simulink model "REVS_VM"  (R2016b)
settings: Solver=ode3  StartTime=REVS.sim_start_time_secs  StopTime=Inf  FixedStep=REVS.sim_step_time_secs  MaxStep=REVS.sim_step_time_secs  EnableMultiTasking=on
StopFcn:
  | postproc_datalog;
  | postproc_audit;
  | postproc_result;
model workspace (MATLAB code in the model file):
  other statements: REVS_setup_variants
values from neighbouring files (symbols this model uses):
  accessory = class_accessory_data    [class_test_data.m]
  battery = class_battery_data    [class_accessory_data.m]    (also in class_REVS_electric.m = class_REVS_battery)
  brake = struct(	'max_torque_Nm',[], 						'proportion_norm',1.0, 						'inertia_kgm2',0.0)    [class_REVS_drive_axle.m]
  engine = class_engine_data    [class_test_data.m]
  final_drive = struct(	'gear_ratio',[], 								'efficiency_norm',[], 								'inertia_kgm2',[] )    [class_REVS_drive_axle.m]
  gear = class_REVS_gearbox    [class_REVS_AT_transmission.m]
  tire = struct(	'radius_m',[], 						'rolling_resistance_coefficient',0, 						'vehicle_weight_norm',1.0,  						'wheel_slip_torque_Nm',[],  						'inertia_kgm2',0.0)    [class_REVS_drive_axle.m]
  torque_converter = class_REVS_torque_converter    [class_REVS_AT_transmission.m]
  transmission = class_transmission_data    [class_test_data.m]
  vehicle = class_vehicle_data    [class_test_data.m]
undefined symbols (not defined in the file or in its folder): alternator, ambient, controls, convert, DelayTimeSecs, drive_cycle, driver, electric, gear_strategy, InitialCondition, InitialValue, LoadSource, LookupStructure, MultiplyPosInputs, Normalize, NumPhases, REVS, SpeedSource, starter, tableshift, UpperSaturationLimit, Value, VerboseLevel, VerboseSignal
libraries: simulink x153
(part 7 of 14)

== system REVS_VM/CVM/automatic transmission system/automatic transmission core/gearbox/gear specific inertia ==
  engage : Inport
  cmd_gear_num : Inport  Port=2
  iner_spd_out_radps : Inport  Port=3
  1-D Lookup Table : Lookup_n-D  NumberOfTableDimensions=1  BreakpointsForDimension1=gear.number  Table=gear.inertia_kgm2  InternalRulePriority=Speed  RndMeth=Simplest
  Derivative : Derivative
  Detect Decrease : simulink/Logic and Bit Operations/Detect Decrease  vinit=0.0  InputProcessing=Inherited  OutDataTypeStr=boolean
  Gain : Gain  Gain=.5/1000
  Gain1 : Gain  Gain=0.5
  Inertia Mech E&P Nm radps : Subsystem
  Memory : Memory
  Memory1 : Memory
  Product : Product  Inputs=3
  Product1 : Product
  Product4 : Product
  Product5 : Product
  Saturation : Saturate  UpperLimit=inf  LowerLimit=0
  Sum : Sum  Inputs=|++
  inertia KE loss : Subsystem
  iner_trq_out_Nm : Outport
  iner_out_kgm2 : Outport  Port=2
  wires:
  cmd_gear_num/1 -> 1-D Lookup Table/1
  Memory1/1 -> Sum/2
  Sum/1 -> inertia KE loss/1(Var), Memory1/1
  Gain1/1 -> Inertia Mech E&P Nm radps/1(trq_Nm)
  Product5/1 -> Gain1/1, iner_trq_out_Nm/1
  Product4/1 -> iner_out_kgm2/1, Product/1, Derivative/1
  iner_spd_out_radps/1 -> Product5/2, Inertia Mech E&P Nm radps/2(spd_radps), Product/2, Product/3
  Memory/1 -> Product1/1
  Detect Decrease/1 -> Product1/2
  Product/1 -> Gain/1
  Gain/1 -> Memory/1
  engage/1 -> Product4/1, Detect Decrease/1
  Derivative/1 -> Saturation/1
  Saturation/1 -> Product5/1
  1-D Lookup Table/1 -> Product4/2
  Product1/1 -> Sum/1

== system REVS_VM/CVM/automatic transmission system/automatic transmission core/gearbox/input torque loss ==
  bus : Inport
  Bus Selector : BusSelector  OutputSignals=gb.gb_cmd_gear,gb_spd_in_radps,ctrl.gb_line_press_bar
  Lookup : Lookup_n-D  NumberOfTableDimensions=10  BreakpointsForDimension1=LookupStructure.axis_1.breakpoints  BreakpointsForDimension2=LookupStructure.axis_2.breakpoints  BreakpointsForDimension3=LookupStructure.axis_3.breakpoints  BreakpointsForDimension4=LookupStructure.axis_4.breakpoints  BreakpointsForDimension5=LookupStructure.axis_5.breakpoints  BreakpointsForDimension6=LookupStructure.axis_6.breakpoints  BreakpointsForDimension7=LookupStructure.axis_7.breakpoints  BreakpointsForDimension8=LookupStructure.axis_8.breakpoints  BreakpointsForDimension9=LookupStructure.axis_9.breakpoints  BreakpointsForDimension10=LookupStructure.axis_10.breakpoints  IndexSearchMethod=Linear search  BeginIndexSearchUsingPreviousIndexResult=on  Table=LookupStructure.table  InternalRulePriority=Speed  RndMeth=Simplest  SupportTunableTableSize=on  MaximumIndicesForEachDimension=LookupStructure.table_size
  out : Outport
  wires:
  bus/1 -> Bus Selector/1
  Lookup/1 -> out/1

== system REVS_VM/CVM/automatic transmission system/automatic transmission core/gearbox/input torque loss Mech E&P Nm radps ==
  trq_Nm : Inport
  spd_radps : Inport  Port=2
  Compare To Constant : simulink/Logic and Bit Operations/Compare To Constant  relop=>=  const=1  OutDataTypeStr=boolean
  Constant : Constant  Value=VerboseSignal
  Subsystem : Subsystem
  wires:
  trq_Nm/1 -> Subsystem/1(trq_Nm)
  spd_radps/1 -> Subsystem/2(spd_radps)
  Compare To Constant/1 -> Subsystem/Enable
  Constant/1 -> Compare To Constant/1

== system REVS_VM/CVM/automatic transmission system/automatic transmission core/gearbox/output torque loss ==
  bus : Inport
  Bus Selector : BusSelector  OutputSignals=gb.gb_cmd_gear,gb_spd_in_radps,ctrl.gb_line_press_bar
  Lookup : Lookup_n-D  NumberOfTableDimensions=10  BreakpointsForDimension1=LookupStructure.axis_1.breakpoints  BreakpointsForDimension2=LookupStructure.axis_2.breakpoints  BreakpointsForDimension3=LookupStructure.axis_3.breakpoints  BreakpointsForDimension4=LookupStructure.axis_4.breakpoints  BreakpointsForDimension5=LookupStructure.axis_5.breakpoints  BreakpointsForDimension6=LookupStructure.axis_6.breakpoints  BreakpointsForDimension7=LookupStructure.axis_7.breakpoints  BreakpointsForDimension8=LookupStructure.axis_8.breakpoints  BreakpointsForDimension9=LookupStructure.axis_9.breakpoints  BreakpointsForDimension10=LookupStructure.axis_10.breakpoints  IndexSearchMethod=Linear search  BeginIndexSearchUsingPreviousIndexResult=on  Table=LookupStructure.table  DiagnosticForOutOfRangeInput=Warning  InternalRulePriority=Speed  RndMeth=Simplest  SupportTunableTableSize=on  MaximumIndicesForEachDimension=LookupStructure.table_size
  out : Outport
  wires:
  bus/1 -> Bus Selector/1
  Lookup/1 -> out/1

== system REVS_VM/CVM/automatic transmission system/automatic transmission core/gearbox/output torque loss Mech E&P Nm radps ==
  trq_Nm : Inport
  spd_radps : Inport  Port=2
  Compare To Constant : simulink/Logic and Bit Operations/Compare To Constant  relop=>=  const=1  OutDataTypeStr=boolean
  Constant : Constant  Value=VerboseSignal
  Subsystem : Subsystem
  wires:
  trq_Nm/1 -> Subsystem/1(trq_Nm)
  spd_radps/1 -> Subsystem/2(spd_radps)
  Compare To Constant/1 -> Subsystem/Enable
  Constant/1 -> Compare To Constant/1

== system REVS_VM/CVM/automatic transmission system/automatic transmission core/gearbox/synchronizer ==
  engage : Inport
  sync_trq_in_Nm : Inport  Port=2
  sync_iner_in_kgm2 : Inport  Port=3
  sync_spd_out_radps : Inport  Port=4
  " clutch input speed integrator (integrate when slipping)" : Integrator  ExternalReset=falling  InitialConditionSource=external  LimitOutput=on  UpperSaturationLimit=Inf  LowerSaturationLimit=0
  Clutch Speed Disengaged : Switch  Threshold=1
  IC1 : InitialCondition  Value=0
  Product : Product
  Product2 : Product  Inputs=*/
  Product3 : Product
  Subsystem : Subsystem
  Sum1 : Sum  Inputs=+-|
  Sum2 : Sum  Inputs=+-|
  Torque SW : Switch  Threshold=1
  engage target speed calc : Subsystem
  synchro limit torque : Subsystem
  to datalog with base name : Subsystem
  to datalog with base name1 : Subsystem
  to datalog with base name2 : Subsystem
  sync_trq_out_Nm : Outport
  sync_iner_out_kgm2 : Outport  Port=2
  sync_spd_in_radps : Outport  Port=3
  sync_lockup : Outport  Port=4
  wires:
  Product2/1 -> " clutch input speed integrator (integrate when slipping)"/1
  synchro limit torque/1(lim_transmit_torque_Nm) -> Sum1/2, to datalog with base name1/1(Var), Torque SW/3
  Product3/1 -> sync_iner_out_kgm2/1
  Torque SW/1 -> sync_trq_out_Nm/1
  Product/1 -> Sum2/2, to datalog with base name2/1(Var)
  " clutch input speed integrator (integrate when slipping)"/1 -> Clutch Speed Disengaged/3
  sync_trq_in_Nm/1 -> Sum2/1, Sum1/1, Torque SW/1
  IC1/1 -> " clutch input speed integrator (integrate when slipping)"/3
  sync_iner_in_kgm2/1 -> Product3/1, Product/2, Product2/2
  engage target speed calc/1(engage_accel_radps2) -> Product/1
  Sum2/1 -> synchro limit torque/2("req_transmit_torque_Nm ")
  Sum1/1 -> Product2/1
  engage/1 -> engage target speed calc/1(engage), Subsystem/1(engage), synchro limit torque/1(engage)
  sync_spd_out_radps/1 -> Subsystem/2(spd_out), synchro limit torque/4(output_speed_radps), IC1/1, engage target speed calc/2(final_spd_radps), Clutch Speed Disengaged/1
  Clutch Speed Disengaged/1 -> sync_spd_in_radps/1, synchro limit torque/3(input_speed_radps), Subsystem/3(spd_in), engage target speed calc/3(current_spd_radps)
  Subsystem/1(lockup) -> to datalog with base name/1(Var), " clutch input speed integrator (integrate when slipping)"/2, sync_lockup/1, Clutch Speed Disengaged/2, Product3/2, Torque SW/2

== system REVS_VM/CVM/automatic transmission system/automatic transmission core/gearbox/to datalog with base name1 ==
  Var : Inport
  Constant : Constant  Value=VerboseSignal
  Constant1 : Constant  Value=VerboseLevel
  Relational Operator : RelationalOperator  OutDataTypeStr=boolean  ZeroCross=off
  Subsystem : Subsystem
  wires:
  Constant1/1 -> Relational Operator/2
  Relational Operator/1 -> Subsystem/Enable
  Constant/1 -> Relational Operator/1
  Var/1 -> Subsystem/1(Var)

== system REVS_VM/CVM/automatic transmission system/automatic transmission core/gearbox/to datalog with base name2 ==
  Var : Inport
  Constant : Constant  Value=VerboseSignal
  Constant1 : Constant  Value=VerboseLevel
  Relational Operator : RelationalOperator  OutDataTypeStr=boolean  ZeroCross=off
  Subsystem : Subsystem
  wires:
  Constant1/1 -> Relational Operator/2
  Relational Operator/1 -> Subsystem/Enable
  Constant/1 -> Relational Operator/1
  Var/1 -> Subsystem/1(Var)

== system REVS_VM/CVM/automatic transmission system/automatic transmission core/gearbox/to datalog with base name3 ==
  Var : Inport
  Constant : Constant  Value=VerboseSignal
  Constant1 : Constant  Value=VerboseLevel
  Relational Operator : RelationalOperator  OutDataTypeStr=boolean  ZeroCross=off
  Subsystem : Subsystem
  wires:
  Constant1/1 -> Relational Operator/2
  Relational Operator/1 -> Subsystem/Enable
  Constant/1 -> Relational Operator/1
  Var/1 -> Subsystem/1(Var)

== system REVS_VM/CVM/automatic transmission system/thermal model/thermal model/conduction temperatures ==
  bus : Inport
  Bus Selector : BusSelector  OutputSignals=signal1,bus.signal2  OutputAsBus=on
  Reshape : Reshape
  out : Outport
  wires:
  Bus Selector/1 -> Reshape/1
  bus/1 -> Bus Selector/1
  Reshape/1 -> out/1

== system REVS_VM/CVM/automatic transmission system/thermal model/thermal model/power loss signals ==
  bus : Inport
  Bus Creator : BusCreator  Inputs=10
  Bus Creator1 : BusCreator  Inputs=2
  Bus Selector : BusSelector  OutputSignals=var_sigs.var_sig1  OutputAsBus=on
  Data Type Conversion : DataTypeConversion  OutDataTypeStr=double
  Display : Display
  Fcn : Fcn
  Variable {1..10} (10 alike) : Constant  Value=nan
  out : Outport
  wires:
  Data Type Conversion/1 -> Fcn/1
  Bus Selector/1 -> Data Type Conversion/1, Display/1
  Bus Creator1/1 -> Bus Selector/1
  Fcn/1 -> out/1
  bus/1 -> Bus Creator1/1  "system_bus"
  Bus Creator/1 -> Bus Creator1/2  "var_sigs"
  Variable 1/1 -> Bus Creator/1  "var_sig1"
  Variable 2/1 -> Bus Creator/2  "var_sig2"
  Variable 3/1 -> Bus Creator/3  "var_sig3"
  Variable 4/1 -> Bus Creator/4  "var_sig4"
  Variable 5/1 -> Bus Creator/5  "var_sig5"
  Variable 6/1 -> Bus Creator/6  "var_sig6"
  Variable 7/1 -> Bus Creator/7  "var_sig7"
  Variable 8/1 -> Bus Creator/8  "var_sig8"
  Variable 9/1 -> Bus Creator/9  "var_sig9"
  Variable 10/1 -> Bus Creator/10  "var_sig10"

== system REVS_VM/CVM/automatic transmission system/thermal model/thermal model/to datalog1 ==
  Var : Inport
  Constant : Constant  Value=VerboseSignal
  Constant1 : Constant  Value=VerboseLevel
  Relational Operator : RelationalOperator  OutDataTypeStr=boolean  ZeroCross=off
  Subsystem : Subsystem
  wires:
  Constant1/1 -> Relational Operator/2
  Constant/1 -> Relational Operator/1
  Relational Operator/1 -> Subsystem/Enable
  Var/1 -> Subsystem/1(In1)

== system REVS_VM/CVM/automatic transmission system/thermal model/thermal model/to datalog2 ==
  Var : Inport
  Constant : Constant  Value=VerboseSignal
  Constant1 : Constant  Value=VerboseLevel
  Relational Operator : RelationalOperator  OutDataTypeStr=boolean  ZeroCross=off
  Subsystem : Subsystem
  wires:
  Constant1/1 -> Relational Operator/2
  Constant/1 -> Relational Operator/1
  Relational Operator/1 -> Subsystem/Enable
  Var/1 -> Subsystem/1(In1)

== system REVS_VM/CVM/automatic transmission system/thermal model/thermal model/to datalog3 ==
  Var : Inport
  Constant : Constant  Value=VerboseSignal
  Constant1 : Constant  Value=VerboseLevel
  Relational Operator : RelationalOperator  OutDataTypeStr=boolean  ZeroCross=off
  Subsystem : Subsystem
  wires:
  Constant1/1 -> Relational Operator/2
  Constant/1 -> Relational Operator/1
  Relational Operator/1 -> Subsystem/Enable
  Var/1 -> Subsystem/1(In1)

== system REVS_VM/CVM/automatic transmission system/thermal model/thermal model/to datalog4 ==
  Var : Inport
  Constant : Constant  Value=VerboseSignal
  Constant1 : Constant  Value=VerboseLevel
  Relational Operator : RelationalOperator  OutDataTypeStr=boolean  ZeroCross=off
  Subsystem : Subsystem
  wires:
  Constant1/1 -> Relational Operator/2
  Constant/1 -> Relational Operator/1
  Relational Operator/1 -> Subsystem/Enable
  Var/1 -> Subsystem/1(In1)

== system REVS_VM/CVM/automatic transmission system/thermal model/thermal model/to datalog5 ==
  Var : Inport
  Constant : Constant  Value=VerboseSignal
  Constant1 : Constant  Value=VerboseLevel
  Relational Operator : RelationalOperator  OutDataTypeStr=boolean  ZeroCross=off
  Subsystem : Subsystem
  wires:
  Constant1/1 -> Relational Operator/2
  Constant/1 -> Relational Operator/1
  Relational Operator/1 -> Subsystem/Enable
  Var/1 -> Subsystem/1(In1)

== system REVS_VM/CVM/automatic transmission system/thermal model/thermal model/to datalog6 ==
  Var : Inport
  Constant : Constant  Value=VerboseSignal
  Constant1 : Constant  Value=VerboseLevel
  Relational Operator : RelationalOperator  OutDataTypeStr=boolean  ZeroCross=off
  Subsystem : Subsystem
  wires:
  Constant1/1 -> Relational Operator/2
  Constant/1 -> Relational Operator/1
  Relational Operator/1 -> Subsystem/Enable
  Var/1 -> Subsystem/1(In1)

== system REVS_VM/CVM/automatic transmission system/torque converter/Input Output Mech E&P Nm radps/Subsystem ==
  trq_in_Nm : Inport
  spd_in_radps : Inport  Port=2
  iner_in_kgm2 : Inport  Port=3
  trq_out_Nm : Inport  Port=4
  spd_out_radps : Inport  Port=5
  iner_out_kgm2 : Inport  Port=6
  Enable : EnablePort  ZeroCross=off
  Input Mech E&P Nm radps : Subsystem
  Loss_KJ_to_workspace : ToWorkspace  VariableName=audit__mech__torque_converter__loss_kJ  SampleTime=-1
  Output Mech E&P Nm radps : Subsystem
  Pos : Saturate  UpperLimit=Inf  LowerLimit=0  ZeroCross=off
  Pos2 : Saturate  UpperLimit=Inf  LowerLimit=0  ZeroCross=off
  Sum : Sum  Inputs=|+-
  Sum1 : Sum  Inputs=-+|
  Sum2 : Sum
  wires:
  Pos2/1 -> Sum2/2
  Pos/1 -> Sum2/1
  trq_in_Nm/1 -> Input Mech E&P Nm radps/1(" trq_Nm")
  spd_in_radps/1 -> Input Mech E&P Nm radps/2(spd_radps)
  trq_out_Nm/1 -> Output Mech E&P Nm radps/1(" trq_Nm")
  spd_out_radps/1 -> Output Mech E&P Nm radps/2(spd_radps)
  iner_in_kgm2/1 -> Input Mech E&P Nm radps/3(iner_kgm2)
  iner_out_kgm2/1 -> Output Mech E&P Nm radps/3(iner_kgm2)
  Input Mech E&P Nm radps/1(pos_kJ) -> Sum/1
  Output Mech E&P Nm radps/1(pos_kJ) -> Sum/2
  Output Mech E&P Nm radps/2(neg_kJ) -> Sum1/2
  Input Mech E&P Nm radps/2(neg_kJ) -> Sum1/1
  Sum/1 -> Pos/1
  Sum1/1 -> Pos2/1
  Sum2/1 -> Loss_KJ_to_workspace/1

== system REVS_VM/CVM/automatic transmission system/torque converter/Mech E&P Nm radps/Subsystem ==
  trq_Nm : Inport
  spd_radps : Inport  Port=2
  Enable : EnablePort  ZeroCross=off
  Mech Energy Nm radps : Subsystem  TreatAsAtomicUnit=on
  energy_to_workspace : ToWorkspace  VariableName=audit__mech__torque_converter__pumploss_kJ  SampleTime=-1
  neg_energy_to_workspace : ToWorkspace  VariableName=audit__mech__torque_converter__pumploss_neg_kJ  SampleTime=-1
  pos_energy_to_workspace : ToWorkspace  VariableName=audit__mech__torque_converter__pumploss_pos_kJ  SampleTime=-1
  power_to_workspace : ToWorkspace  VariableName=audit__mech__torque_converter__pumploss_kW  SampleTime=-1
  speed_to_workspace : ToWorkspace  VariableName=audit__mech__torque_converter__pumploss_radps  SampleTime=-1
  torque_to_workspace : ToWorkspace  VariableName=audit__mech__torque_converter__pumploss_Nm  SampleTime=-1
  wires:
  Mech Energy Nm radps/1("total_kJ ") -> energy_to_workspace/1
  Mech Energy Nm radps/4(pwr_kW) -> power_to_workspace/1
  Mech Energy Nm radps/2("pos_kJ ") -> pos_energy_to_workspace/1
  Mech Energy Nm radps/3(neg_kJ) -> neg_energy_to_workspace/1
  trq_Nm/1 -> torque_to_workspace/1, Mech Energy Nm radps/1(trq_Nm)
  spd_radps/1 -> speed_to_workspace/1, Mech Energy Nm radps/2(spd_radps)

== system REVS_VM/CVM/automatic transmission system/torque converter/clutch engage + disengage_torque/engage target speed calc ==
  engage : Inport
  final_spd_radps : Inport  Port=2
  current_spd_radps : Inport  Port=3
  Compare To Zero : simulink/Logic and Bit Operations/Compare To Zero  relop=>  OutDataTypeStr=boolean
  Fcn : Fcn  Expr=5*(1-u)^3 + .05
  Product1 : Product  Inputs=**//
  Sum2 : Sum  Inputs=|+-
  engage duration : Constant  Value=Value
  engage_accel_radps2 : Outport
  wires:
  current_spd_radps/1 -> Sum2/2
  Product1/1 -> engage_accel_radps2/1
  final_spd_radps/1 -> Sum2/1
  engage/1 -> Fcn/1, Compare To Zero/1
  Compare To Zero/1 -> Product1/1
  engage duration/1 -> Product1/4
  Sum2/1 -> Product1/2
  Fcn/1 -> Product1/3

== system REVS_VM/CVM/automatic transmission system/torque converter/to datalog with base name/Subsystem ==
  Var : Inport
  Enable : EnablePort
  To Workspace : ToWorkspace  VariableName=datalog__torque_converter__speed_ratio  SampleTime=-1
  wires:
  Var/1 -> To Workspace/1

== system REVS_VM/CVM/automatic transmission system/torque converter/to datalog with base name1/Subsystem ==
  Var : Inport
  Enable : EnablePort
  To Workspace : ToWorkspace  VariableName=datalog__torque_converter__torque_ratio  SampleTime=-1
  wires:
  Var/1 -> To Workspace/1

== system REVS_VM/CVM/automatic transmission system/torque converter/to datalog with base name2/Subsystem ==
  Var : Inport
  Enable : EnablePort
  To Workspace : ToWorkspace  VariableName=datalog__torque_converter__k_factor_rpmpsqrtNm  SampleTime=-1
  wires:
  Var/1 -> To Workspace/1

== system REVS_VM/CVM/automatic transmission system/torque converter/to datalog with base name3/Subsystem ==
  Var : Inport
  Enable : EnablePort
  To Workspace : ToWorkspace  VariableName=datalog__torque_converter__tcc_engage_norm  SampleTime=-1
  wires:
  Var/1 -> To Workspace/1

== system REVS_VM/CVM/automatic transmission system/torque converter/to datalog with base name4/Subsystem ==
  Var : Inport
  Enable : EnablePort
  To Workspace : ToWorkspace  VariableName=datalog__torque_converter__hydrodynamic_load_Nm  SampleTime=-1
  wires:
  Var/1 -> To Workspace/1

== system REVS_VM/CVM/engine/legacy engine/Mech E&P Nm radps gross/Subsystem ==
  " trq_Nm" : Inport
  spd_radps : Inport  Port=2
  iner_kgm2 : Inport  Port=3
  Enable : EnablePort  ZeroCross=off
  KE_to_workspace : ToWorkspace  VariableName=audit__mech__engine__crankshaft_gross_KE_kJ  SampleTime=-1
  Mech Energy Nm radps : Subsystem  TreatAsAtomicUnit=on
  Mult : Product  Inputs=**
  Square : Math  Operator=square
  energy_to_workspace : ToWorkspace  VariableName=audit__mech__engine__crankshaft_gross_kJ  SampleTime=-1
  inertia_to_workspace : ToWorkspace  VariableName=audit__mech__engine__crankshaft_gross_kgm2  SampleTime=-1
  neg_energy_to_workspace : ToWorkspace  VariableName=audit__mech__engine__crankshaft_gross_neg_kJ  SampleTime=-1
  one half : Gain  Gain=0.5/1000
  pos_energy_to_workspace : ToWorkspace  VariableName=audit__mech__engine__crankshaft_gross_pos_kJ  SampleTime=-1
  power_to_workspace : ToWorkspace  VariableName=audit__mech__engine__crankshaft_gross_kW  SampleTime=-1
  speed_to_workspace : ToWorkspace  VariableName=audit__mech__engine__crankshaft_gross_radps  SampleTime=-1
  torque_to_workspace : ToWorkspace  VariableName=audit__mech__engine__crankshaft_gross_Nm  SampleTime=-1
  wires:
  " trq_Nm"/1 -> torque_to_workspace/1, Mech Energy Nm radps/1(trq_Nm)
  spd_radps/1 -> Square/1, speed_to_workspace/1, Mech Energy Nm radps/2(spd_radps)
  iner_kgm2/1 -> Mult/2, inertia_to_workspace/1
  Mech Energy Nm radps/1("total_kJ ") -> energy_to_workspace/1
  Mech Energy Nm radps/4(pwr_kW) -> power_to_workspace/1
  Mech Energy Nm radps/2("pos_kJ ") -> pos_energy_to_workspace/1
  Mech Energy Nm radps/3(neg_kJ) -> neg_energy_to_workspace/1
  one half/1 -> KE_to_workspace/1
  Square/1 -> Mult/1
  Mult/1 -> one half/1

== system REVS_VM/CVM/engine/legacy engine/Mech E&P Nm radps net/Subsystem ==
  " trq_Nm" : Inport
  spd_radps : Inport  Port=2
  iner_kgm2 : Inport  Port=3
  Enable : EnablePort  ZeroCross=off
  KE_to_workspace : ToWorkspace  VariableName=audit__mech__engine__crankshaft_KE_kJ  SampleTime=-1
  Mech Energy Nm radps : Subsystem  TreatAsAtomicUnit=on
  Mult : Product  Inputs=**
  Square : Math  Operator=square
  energy_to_workspace : ToWorkspace  VariableName=audit__mech__engine__crankshaft_kJ  SampleTime=-1
  inertia_to_workspace : ToWorkspace  VariableName=audit__mech__engine__crankshaft_kgm2  SampleTime=-1
  neg_energy_to_workspace : ToWorkspace  VariableName=audit__mech__engine__crankshaft_neg_kJ  SampleTime=-1
  one half : Gain  Gain=0.5/1000
  pos_energy_to_workspace : ToWorkspace  VariableName=audit__mech__engine__crankshaft_pos_kJ  SampleTime=-1
  power_to_workspace : ToWorkspace  VariableName=audit__mech__engine__crankshaft_kW  SampleTime=-1
  speed_to_workspace : ToWorkspace  VariableName=audit__mech__engine__crankshaft_radps  SampleTime=-1
  torque_to_workspace : ToWorkspace  VariableName=audit__mech__engine__crankshaft_Nm  SampleTime=-1
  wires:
  " trq_Nm"/1 -> torque_to_workspace/1, Mech Energy Nm radps/1(trq_Nm)
  spd_radps/1 -> Square/1, speed_to_workspace/1, Mech Energy Nm radps/2(spd_radps)
  iner_kgm2/1 -> Mult/2, inertia_to_workspace/1
  Mech Energy Nm radps/1("total_kJ ") -> energy_to_workspace/1
  Mech Energy Nm radps/4(pwr_kW) -> power_to_workspace/1
  Mech Energy Nm radps/2("pos_kJ ") -> pos_energy_to_workspace/1
  Mech Energy Nm radps/3(neg_kJ) -> neg_energy_to_workspace/1
  one half/1 -> KE_to_workspace/1
  Square/1 -> Mult/1
  Mult/1 -> one half/1

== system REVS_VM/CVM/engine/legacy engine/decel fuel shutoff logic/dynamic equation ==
  bus : Inport
  Bus Creator : BusCreator  Inputs=10
  Bus Creator1 : BusCreator  Inputs=2
  Bus Selector : BusSelector  OutputSignals=var_sigs.var_sig1  OutputAsBus=on
  Data Type Conversion : DataTypeConversion  OutDataTypeStr=double
  Display : Display
  Fcn : Fcn
  Variable {1..10} (10 alike) : Constant  Value=nan
  out : Outport
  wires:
  Data Type Conversion/1 -> Fcn/1
  Bus Selector/1 -> Data Type Conversion/1, Display/1
  Bus Creator1/1 -> Bus Selector/1
  Fcn/1 -> out/1
  bus/1 -> Bus Creator1/1  "system_bus"
  Bus Creator/1 -> Bus Creator1/2  "var_sigs"
  Variable 1/1 -> Bus Creator/1  "var_sig1"
  Variable 2/1 -> Bus Creator/2  "var_sig2"
  Variable 3/1 -> Bus Creator/3  "var_sig3"
  Variable 4/1 -> Bus Creator/4  "var_sig4"
  Variable 5/1 -> Bus Creator/5  "var_sig5"
  Variable 6/1 -> Bus Creator/6  "var_sig6"
  Variable 7/1 -> Bus Creator/7  "var_sig7"
  Variable 8/1 -> Bus Creator/8  "var_sig8"
  Variable 9/1 -> Bus Creator/9  "var_sig9"
  Variable 10/1 -> Bus Creator/10  "var_sig10"

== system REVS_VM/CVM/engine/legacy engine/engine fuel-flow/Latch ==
  On : Inport  PortDimensions=1
  Off : Inport  Port=2  PortDimensions=1
  Combinatorial  Logic : CombinatorialLogic  TruthTable=[0;1;0;0;1;1;(tb==2);(tb>=2)]
  Memory2 : Memory  X0=InitialCondition
  Mux : Mux  Inputs=3
  State : Outport  PortDimensions=1
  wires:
  Off/1 -> Mux/2
  On/1 -> Mux/1
  Memory2/1 -> Mux/3
  Mux/1 -> Combinatorial  Logic/1
  Combinatorial  Logic/1 -> State/1, Memory2/1

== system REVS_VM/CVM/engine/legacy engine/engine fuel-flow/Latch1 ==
  On : Inport  PortDimensions=1
  Off : Inport  Port=2  PortDimensions=1
  Combinatorial  Logic : CombinatorialLogic  TruthTable=[0;1;0;0;1;1;(tb==2);(tb>=2)]
  Memory2 : Memory  X0=InitialCondition
  Mux : Mux  Inputs=3
  State : Outport  PortDimensions=1
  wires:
  Off/1 -> Mux/2
  On/1 -> Mux/1
  Memory2/1 -> Mux/3
  Mux/1 -> Combinatorial  Logic/1
  Combinatorial  Logic/1 -> State/1, Memory2/1

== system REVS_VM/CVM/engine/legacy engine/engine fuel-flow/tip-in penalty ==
  bool : Inport
  Constant : Constant  Value=Normalize
  Data Type Conversion2 : DataTypeConversion  OutDataTypeStr=double
  Integrator1 : Integrator  ExternalReset=falling  LimitOutput=on  UpperSaturationLimit=UpperSaturationLimit  LowerSaturationLimit=0
  Switch : Switch  Criteria=u2 > Threshold
  normalize : Gain  Gain=1/UpperSaturationLimit
  out : Outport
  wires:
  Switch/1 -> out/1
  normalize/1 -> Switch/1
  Integrator1/1 -> Switch/3, normalize/1
  Constant/1 -> Switch/2
  bool/1 -> Data Type Conversion2/1
  Data Type Conversion2/1 -> Integrator1/1, Integrator1/2

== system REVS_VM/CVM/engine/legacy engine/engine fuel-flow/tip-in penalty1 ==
  bool : Inport
  Constant : Constant  Value=Normalize
  Data Type Conversion2 : DataTypeConversion  OutDataTypeStr=double
  Integrator1 : Integrator  ExternalReset=falling  LimitOutput=on  UpperSaturationLimit=UpperSaturationLimit  LowerSaturationLimit=0
  Switch : Switch  Criteria=u2 > Threshold
  normalize : Gain  Gain=1/UpperSaturationLimit
  out : Outport
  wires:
  Switch/1 -> out/1
  normalize/1 -> Switch/1
  Integrator1/1 -> Switch/3, normalize/1
  Constant/1 -> Switch/2
  bool/1 -> Data Type Conversion2/1
  Data Type Conversion2/1 -> Integrator1/1, Integrator1/2

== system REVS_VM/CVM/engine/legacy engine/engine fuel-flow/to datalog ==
  Var : Inport
  Constant : Constant  Value=VerboseSignal
  Constant1 : Constant  Value=VerboseLevel
  Relational Operator : RelationalOperator  OutDataTypeStr=boolean  ZeroCross=off
  Subsystem : Subsystem
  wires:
  Constant1/1 -> Relational Operator/2
  Constant/1 -> Relational Operator/1
  Relational Operator/1 -> Subsystem/Enable
  Var/1 -> Subsystem/1(In1)

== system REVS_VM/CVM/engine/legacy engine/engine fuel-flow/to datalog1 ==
  Var : Inport
  Constant : Constant  Value=VerboseSignal
  Constant1 : Constant  Value=VerboseLevel
  Relational Operator : RelationalOperator  OutDataTypeStr=boolean  ZeroCross=off
  Subsystem : Subsystem
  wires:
  Constant1/1 -> Relational Operator/2
  Constant/1 -> Relational Operator/1
  Relational Operator/1 -> Subsystem/Enable
  Var/1 -> Subsystem/1(In1)

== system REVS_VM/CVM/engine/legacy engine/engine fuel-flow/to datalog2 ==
  Var : Inport
  Constant : Constant  Value=VerboseSignal
  Constant1 : Constant  Value=VerboseLevel
  Relational Operator : RelationalOperator  OutDataTypeStr=boolean  ZeroCross=off
  Subsystem : Subsystem
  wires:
  Constant1/1 -> Relational Operator/2
  Constant/1 -> Relational Operator/1
  Relational Operator/1 -> Subsystem/Enable
  Var/1 -> Subsystem/1(In1)

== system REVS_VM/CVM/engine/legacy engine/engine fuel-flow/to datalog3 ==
  Var : Inport
  Constant : Constant  Value=VerboseSignal
  Constant1 : Constant  Value=VerboseLevel
  Relational Operator : RelationalOperator  OutDataTypeStr=boolean  ZeroCross=off
  Subsystem : Subsystem
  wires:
  Constant1/1 -> Relational Operator/2
  Constant/1 -> Relational Operator/1
  Relational Operator/1 -> Subsystem/Enable
  Var/1 -> Subsystem/1(In1)

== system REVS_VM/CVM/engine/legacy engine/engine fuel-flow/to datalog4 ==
  Var : Inport
  Constant : Constant  Value=VerboseSignal
  Constant1 : Constant  Value=VerboseLevel
  Relational Operator : RelationalOperator  OutDataTypeStr=boolean  ZeroCross=off
  Subsystem : Subsystem
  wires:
  Constant1/1 -> Relational Operator/2
  Constant/1 -> Relational Operator/1
  Relational Operator/1 -> Subsystem/Enable
  Var/1 -> Subsystem/1(In1)

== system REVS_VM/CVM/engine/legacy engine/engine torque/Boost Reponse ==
  target_trq_Nm : Inport
  max_trq_Nm : Inport  Port=2
  nat_asp_trq_Nm : Inport  Port=3
  Dynamic Limit Integrator : Subsystem
  Gain2 : Gain  Gain=1/engine.boost_time_constant_secs
  MinMax3 : MinMax  Function=max  Inputs=2  ZeroCross=off
  MinMax4 : MinMax  Inputs=2  ZeroCross=off
  Sum : Sum  Inputs=|+-
  trq_limit_Nm : Outport
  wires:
  Dynamic Limit Integrator/1(Out) -> Sum/2, trq_limit_Nm/1
  MinMax3/1 -> MinMax4/1
  Sum/1 -> Gain2/1
  MinMax4/1 -> Sum/1
  Gain2/1 -> Dynamic Limit Integrator/2(In)
  nat_asp_trq_Nm/1 -> Dynamic Limit Integrator/5(lower), Dynamic Limit Integrator/4(Xo), MinMax3/2
  max_trq_Nm/1 -> Dynamic Limit Integrator/1(upper), MinMax4/2
  target_trq_Nm/1 -> MinMax3/1

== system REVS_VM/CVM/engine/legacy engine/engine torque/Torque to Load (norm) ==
  torque : Inport
  max : Inport  Port=2
  min : Inport  Port=3
  Divide1 : Product  Inputs=*/
  Saturation1 : Saturate  UpperLimit=Inf  LowerLimit=1  ZeroCross=off
  Sum4 : Sum  Inputs=+-
  Sum5 : Sum  Inputs=+-
  load_norm : Outport
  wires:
  max/1 -> Sum4/1
  min/1 -> Sum5/2, Sum4/2
  Divide1/1 -> load_norm/1
  Sum5/1 -> Divide1/1
  torque/1 -> Sum5/1
  Sum4/1 -> Saturation1/1
  Saturation1/1 -> Divide1/2

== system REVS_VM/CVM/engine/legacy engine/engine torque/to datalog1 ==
  Var : Inport
  Constant : Constant  Value=VerboseSignal
  Constant1 : Constant  Value=VerboseLevel
  Relational Operator : RelationalOperator  OutDataTypeStr=boolean  ZeroCross=off
  Subsystem : Subsystem
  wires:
  Constant1/1 -> Relational Operator/2
  Constant/1 -> Relational Operator/1
  Relational Operator/1 -> Subsystem/Enable
  Var/1 -> Subsystem/1(In1)

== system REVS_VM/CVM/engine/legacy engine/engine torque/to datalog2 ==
  Var : Inport
  Constant : Constant  Value=VerboseSignal
  Constant1 : Constant  Value=VerboseLevel
  Relational Operator : RelationalOperator  OutDataTypeStr=boolean  ZeroCross=off
  Subsystem : Subsystem
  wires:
  Constant1/1 -> Relational Operator/2
  Constant/1 -> Relational Operator/1
  Relational Operator/1 -> Subsystem/Enable
  Var/1 -> Subsystem/1(In1)

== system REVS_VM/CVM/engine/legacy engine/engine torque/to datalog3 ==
  Var : Inport
  Constant : Constant  Value=VerboseSignal
  Constant1 : Constant  Value=VerboseLevel
  Relational Operator : RelationalOperator  OutDataTypeStr=boolean  ZeroCross=off
  Subsystem : Subsystem
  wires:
  Constant1/1 -> Relational Operator/2
  Constant/1 -> Relational Operator/1
  Relational Operator/1 -> Subsystem/Enable
  Var/1 -> Subsystem/1(In1)

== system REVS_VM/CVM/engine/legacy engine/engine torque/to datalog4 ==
  Var : Inport
  Constant : Constant  Value=VerboseSignal
  Constant1 : Constant  Value=VerboseLevel
  Relational Operator : RelationalOperator  OutDataTypeStr=boolean  ZeroCross=off
  Subsystem : Subsystem
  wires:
  Constant1/1 -> Relational Operator/2
  Constant/1 -> Relational Operator/1
  Relational Operator/1 -> Subsystem/Enable
  Var/1 -> Subsystem/1(In1)

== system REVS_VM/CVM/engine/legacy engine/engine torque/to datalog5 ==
  Var : Inport
  Constant : Constant  Value=VerboseSignal
  Constant1 : Constant  Value=VerboseLevel
  Relational Operator : RelationalOperator  OutDataTypeStr=boolean  ZeroCross=off
  Subsystem : Subsystem
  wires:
  Constant1/1 -> Relational Operator/2
  Constant/1 -> Relational Operator/1
  Relational Operator/1 -> Subsystem/Enable
  Var/1 -> Subsystem/1(In1)

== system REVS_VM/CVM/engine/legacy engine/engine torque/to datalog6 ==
  Var : Inport
  Constant : Constant  Value=VerboseSignal
  Constant1 : Constant  Value=VerboseLevel
  Relational Operator : RelationalOperator  OutDataTypeStr=boolean  ZeroCross=off
  Subsystem : Subsystem
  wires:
  Constant1/1 -> Relational Operator/2
  Constant/1 -> Relational Operator/1
  Relational Operator/1 -> Subsystem/Enable
  Var/1 -> Subsystem/1(In1)

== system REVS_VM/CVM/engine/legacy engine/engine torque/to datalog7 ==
  Var : Inport
  Constant : Constant  Value=VerboseSignal
  Constant1 : Constant  Value=VerboseLevel
  Relational Operator : RelationalOperator  OutDataTypeStr=boolean  ZeroCross=off
  Subsystem : Subsystem
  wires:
  Constant1/1 -> Relational Operator/2
  Constant/1 -> Relational Operator/1
  Relational Operator/1 -> Subsystem/Enable
  Var/1 -> Subsystem/1(In1)

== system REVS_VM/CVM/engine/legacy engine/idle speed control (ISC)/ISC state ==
  eng_on : Inport
  eng_spd_radps : Inport  Port=2
  Compare To Constant : simulink/Logic and Bit Operations/Compare To Constant  relop=>  const=0.5  OutDataTypeStr=boolean
  Compare To Zero : simulink/Logic and Bit Operations/Compare To Zero  relop===  OutDataTypeStr=boolean
  Data Type Conversion2 : DataTypeConversion
  Latch : Subsystem
  Logical Operator : Logic  AllPortsSameDT=off  OutDataTypeStr=boolean
  Logical Operator1 : Logic  Operator=OR  AllPortsSameDT=off  OutDataTypeStr=boolean
  Relational Operator : RelationalOperator  Operator=>  OutDataTypeStr=boolean
  Relational Operator1 : RelationalOperator  Operator=<  OutDataTypeStr=boolean
  activation_speed_radps : Constant  Value=engine.idle_control_activation_speed_radps
  boolean integrator : Subsystem
  deactivation_speed_radps : Constant  Value=engine.idle_control_deactivation_speed_radps
  state : Outport
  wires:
  Compare To Zero/1 -> Logical Operator1/2
  Relational Operator1/1 -> Logical Operator1/1
  eng_on/1 -> Logical Operator/1, Compare To Zero/1
  Logical Operator/1 -> boolean integrator/1(bool)
  Data Type Conversion2/1 -> state/1
  Latch/1(State) -> Data Type Conversion2/1
  deactivation_speed_radps/1 -> Relational Operator1/2
  Compare To Constant/1 -> Latch/1(On)
  Logical Operator1/1 -> Latch/2(Off)
  activation_speed_radps/1 -> Relational Operator/2
  eng_spd_radps/1 -> Relational Operator/1, Relational Operator1/1
  boolean integrator/1(out) -> Compare To Constant/1
  Relational Operator/1 -> Logical Operator/2

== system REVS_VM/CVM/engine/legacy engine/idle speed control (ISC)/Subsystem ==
  system_bus : Inport
  eng_des_spd_radps : Inport  Port=2
  eng_spd_radps : Inport  Port=3
  ISC_state : Inport  Port=4
  Data Type Conversion : DataTypeConversion
  MinMax : MinMax  Function=max  Inputs=2
  Product1 : Product
  Rate Limiter : RateLimiter  RisingSlewLimit=1/engine.idle_control_ramp_time_secs  FallingSlewLimit=-1/engine.idle_control_ramp_time_secs
  Relational Operator : RelationalOperator  OutDataTypeStr=boolean
  Sum1 : Sum
  Sum3 : Sum
  idle ramp : Product
  running timer : Integrator  ExternalReset=falling
  soft landing offset radps : Constant  Value=engine.idle_control_ramp_radps
  startup flare : Lookup_n-D  NumberOfTableDimensions=1  BreakpointsForDimension1=[0 0.5 1.25 2.25 3.0 3.5]  IndexSearchMethod=Linear search  Table="[0.5 1.1 1.2 1.2  1.1 1.0]"  InterpMethod=Cubic spline  ExtrapMethod=Clip  RndMeth=Simplest
  target idle speed : Subsystem
  target_idle_spd_radps : Outport
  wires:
  Sum1/1 -> target_idle_spd_radps/1
  Data Type Conversion/1 -> Rate Limiter/1
  idle ramp/1 -> Sum1/1
  Sum3/1 -> Relational Operator/2
  Rate Limiter/1 -> idle ramp/2
  soft landing offset radps/1 -> Sum3/1, idle ramp/1
  Relational Operator/1 -> Data Type Conversion/1
  running timer/1 -> startup flare/1
  Product1/1 -> MinMax/2
  MinMax/1 -> Sum3/2, Sum1/2
  target idle speed/1(out) -> Product1/2
  eng_des_spd_radps/1 -> MinMax/1
  startup flare/1 -> Product1/1
  ISC_state/1 -> running timer/1, running timer/2
  eng_spd_radps/1 -> Relational Operator/1
  system_bus/1 -> target idle speed/1(bus)

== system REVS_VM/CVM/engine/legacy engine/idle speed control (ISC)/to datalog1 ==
  Var : Inport
  Constant : Constant  Value=VerboseSignal
  Constant1 : Constant  Value=VerboseLevel
  Relational Operator : RelationalOperator  OutDataTypeStr=boolean  ZeroCross=off
  Subsystem : Subsystem
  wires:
  Constant1/1 -> Relational Operator/2
  Constant/1 -> Relational Operator/1
  Relational Operator/1 -> Subsystem/Enable
  Var/1 -> Subsystem/1(In1)

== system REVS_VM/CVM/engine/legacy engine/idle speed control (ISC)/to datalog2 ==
  Var : Inport
  Constant : Constant  Value=VerboseSignal
  Constant1 : Constant  Value=VerboseLevel
  Relational Operator : RelationalOperator  OutDataTypeStr=boolean  ZeroCross=off
  Subsystem : Subsystem
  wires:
  Constant1/1 -> Relational Operator/2
  Constant/1 -> Relational Operator/1
  Relational Operator/1 -> Subsystem/Enable
  Var/1 -> Subsystem/1(In1)

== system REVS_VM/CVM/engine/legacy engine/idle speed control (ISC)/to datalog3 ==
  Var : Inport
  Constant : Constant  Value=VerboseSignal
  Constant1 : Constant  Value=VerboseLevel
  Relational Operator : RelationalOperator  OutDataTypeStr=boolean  ZeroCross=off
  Subsystem : Subsystem
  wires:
  Constant1/1 -> Relational Operator/2
  Constant/1 -> Relational Operator/1
  Relational Operator/1 -> Subsystem/Enable
  Var/1 -> Subsystem/1(In1)

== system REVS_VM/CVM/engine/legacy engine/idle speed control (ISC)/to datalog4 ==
  Var : Inport
  Constant : Constant  Value=VerboseSignal
  Constant1 : Constant  Value=VerboseLevel
  Relational Operator : RelationalOperator  OutDataTypeStr=boolean  ZeroCross=off
  Subsystem : Subsystem
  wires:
  Constant1/1 -> Relational Operator/2
  Constant/1 -> Relational Operator/1
  Relational Operator/1 -> Subsystem/Enable
  Var/1 -> Subsystem/1(In1)

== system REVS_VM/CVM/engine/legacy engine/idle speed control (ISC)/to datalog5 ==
  Var : Inport
  Constant : Constant  Value=VerboseSignal
  Constant1 : Constant  Value=VerboseLevel
  Relational Operator : RelationalOperator  OutDataTypeStr=boolean  ZeroCross=off
  Subsystem : Subsystem
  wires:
  Constant1/1 -> Relational Operator/2
  Constant/1 -> Relational Operator/1
  Relational Operator/1 -> Subsystem/Enable
  Var/1 -> Subsystem/1(In1)

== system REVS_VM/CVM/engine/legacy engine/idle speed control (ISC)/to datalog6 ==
  Var : Inport
  Constant : Constant  Value=VerboseSignal
  Constant1 : Constant  Value=VerboseLevel
  Relational Operator : RelationalOperator  OutDataTypeStr=boolean  ZeroCross=off
  Subsystem : Subsystem
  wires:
  Constant1/1 -> Relational Operator/2
  Constant/1 -> Relational Operator/1
  Relational Operator/1 -> Subsystem/Enable
  Var/1 -> Subsystem/1(In1)

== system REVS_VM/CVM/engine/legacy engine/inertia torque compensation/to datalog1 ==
  Var : Inport
  Constant : Constant  Value=VerboseSignal
  Constant1 : Constant  Value=VerboseLevel
  Relational Operator : RelationalOperator  OutDataTypeStr=boolean  ZeroCross=off
  Subsystem : Subsystem
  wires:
  Constant1/1 -> Relational Operator/2
  Constant/1 -> Relational Operator/1
  Relational Operator/1 -> Subsystem/Enable
  Var/1 -> Subsystem/1(In1)

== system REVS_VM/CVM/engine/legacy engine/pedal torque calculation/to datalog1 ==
  Var : Inport
  Constant : Constant  Value=VerboseSignal
  Constant1 : Constant  Value=VerboseLevel
  Relational Operator : RelationalOperator  OutDataTypeStr=boolean  ZeroCross=off
  Subsystem : Subsystem
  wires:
  Constant1/1 -> Relational Operator/2
  Constant/1 -> Relational Operator/1
  Relational Operator/1 -> Subsystem/Enable
  Var/1 -> Subsystem/1(In1)

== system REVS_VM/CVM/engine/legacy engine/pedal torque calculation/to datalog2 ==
  Var : Inport
  Constant : Constant  Value=VerboseSignal
  Constant1 : Constant  Value=VerboseLevel
  Relational Operator : RelationalOperator  OutDataTypeStr=boolean  ZeroCross=off
  Subsystem : Subsystem
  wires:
  Constant1/1 -> Relational Operator/2
  Constant/1 -> Relational Operator/1
  Relational Operator/1 -> Subsystem/Enable
  Var/1 -> Subsystem/1(In1)

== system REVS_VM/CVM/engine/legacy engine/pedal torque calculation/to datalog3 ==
  Var : Inport
  Constant : Constant  Value=VerboseSignal
  Constant1 : Constant  Value=VerboseLevel
  Relational Operator : RelationalOperator  OutDataTypeStr=boolean  ZeroCross=off
  Subsystem : Subsystem
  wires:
  Constant1/1 -> Relational Operator/2
  Constant/1 -> Relational Operator/1
  Relational Operator/1 -> Subsystem/Enable
  Var/1 -> Subsystem/1(In1)

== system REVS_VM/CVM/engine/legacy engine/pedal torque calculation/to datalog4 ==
  Var : Inport
  Constant : Constant  Value=VerboseSignal
  Constant1 : Constant  Value=VerboseLevel
  Relational Operator : RelationalOperator  OutDataTypeStr=boolean  ZeroCross=off
  Subsystem : Subsystem
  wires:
  Constant1/1 -> Relational Operator/2
  Constant/1 -> Relational Operator/1
  Relational Operator/1 -> Subsystem/Enable
  Var/1 -> Subsystem/1(In1)

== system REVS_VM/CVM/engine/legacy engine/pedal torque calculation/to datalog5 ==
  Var : Inport
  Constant : Constant  Value=VerboseSignal
  Constant1 : Constant  Value=VerboseLevel
  Relational Operator : RelationalOperator  OutDataTypeStr=boolean  ZeroCross=off
  Subsystem : Subsystem
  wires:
  Constant1/1 -> Relational Operator/2
  Constant/1 -> Relational Operator/1
  Relational Operator/1 -> Subsystem/Enable
  Var/1 -> Subsystem/1(In1)

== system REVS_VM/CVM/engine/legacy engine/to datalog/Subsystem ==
  In1 : Inport
  Enable : EnablePort
  To Workspace : ToWorkspace  VariableName=datalog__engine__fuel_rate_gps  SampleTime=-1
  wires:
  In1/1 -> To Workspace/1

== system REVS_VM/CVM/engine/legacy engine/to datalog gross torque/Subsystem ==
  In1 : Inport
  Enable : EnablePort
  To Workspace : ToWorkspace  VariableName=datalog__engine__crankshaft_gross_torque_Nm  SampleTime=-1
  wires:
  In1/1 -> To Workspace/1

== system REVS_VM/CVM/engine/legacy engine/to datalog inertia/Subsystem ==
  In1 : Inport
  Enable : EnablePort
  To Workspace : ToWorkspace  VariableName=datalog__engine__crankshaft_gross_inertia_kgm2  SampleTime=-1
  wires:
  In1/1 -> To Workspace/1

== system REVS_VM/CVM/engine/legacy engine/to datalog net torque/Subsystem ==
  In1 : Inport
  Enable : EnablePort
  To Workspace : ToWorkspace  VariableName=datalog__engine__crankshaft_torque_Nm  SampleTime=-1
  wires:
  In1/1 -> To Workspace/1

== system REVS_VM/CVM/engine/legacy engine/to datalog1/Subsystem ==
  In1 : Inport
  Enable : EnablePort
  To Workspace : ToWorkspace  VariableName=datalog__engine__fuel_consumed_g  SampleTime=-1
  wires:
  In1/1 -> To Workspace/1

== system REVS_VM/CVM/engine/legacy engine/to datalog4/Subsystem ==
  In1 : Inport
  Enable : EnablePort
  To Workspace : ToWorkspace  VariableName=datalog__engine__crankshaft_speed_radps  SampleTime=-1
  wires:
  In1/1 -> To Workspace/1

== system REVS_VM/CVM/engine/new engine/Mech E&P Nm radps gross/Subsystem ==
  " trq_Nm" : Inport
  spd_radps : Inport  Port=2
  iner_kgm2 : Inport  Port=3
  Enable : EnablePort  ZeroCross=off
  KE_to_workspace : ToWorkspace  VariableName=audit__mech__engine__crankshaft_gross_KE_kJ  SampleTime=-1
  Mech Energy Nm radps : Subsystem  TreatAsAtomicUnit=on
  Mult : Product  Inputs=**
  Square : Math  Operator=square
  energy_to_workspace : ToWorkspace  VariableName=audit__mech__engine__crankshaft_gross_kJ  SampleTime=-1
  inertia_to_workspace : ToWorkspace  VariableName=audit__mech__engine__crankshaft_gross_kgm2  SampleTime=-1
  neg_energy_to_workspace : ToWorkspace  VariableName=audit__mech__engine__crankshaft_gross_neg_kJ  SampleTime=-1
  one half : Gain  Gain=0.5/1000
  pos_energy_to_workspace : ToWorkspace  VariableName=audit__mech__engine__crankshaft_gross_pos_kJ  SampleTime=-1
  power_to_workspace : ToWorkspace  VariableName=audit__mech__engine__crankshaft_gross_kW  SampleTime=-1
  speed_to_workspace : ToWorkspace  VariableName=audit__mech__engine__crankshaft_gross_radps  SampleTime=-1
  torque_to_workspace : ToWorkspace  VariableName=audit__mech__engine__crankshaft_gross_Nm  SampleTime=-1
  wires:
  " trq_Nm"/1 -> torque_to_workspace/1, Mech Energy Nm radps/1(trq_Nm)
  spd_radps/1 -> Square/1, speed_to_workspace/1, Mech Energy Nm radps/2(spd_radps)
  iner_kgm2/1 -> Mult/2, inertia_to_workspace/1
  Mech Energy Nm radps/1("total_kJ ") -> energy_to_workspace/1
  Mech Energy Nm radps/4(pwr_kW) -> power_to_workspace/1
  Mech Energy Nm radps/2("pos_kJ ") -> pos_energy_to_workspace/1
  Mech Energy Nm radps/3(neg_kJ) -> neg_energy_to_workspace/1
  one half/1 -> KE_to_workspace/1
  Square/1 -> Mult/1
  Mult/1 -> one half/1

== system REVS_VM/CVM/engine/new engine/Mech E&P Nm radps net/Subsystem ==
  " trq_Nm" : Inport
  spd_radps : Inport  Port=2
  iner_kgm2 : Inport  Port=3
  Enable : EnablePort  ZeroCross=off
  KE_to_workspace : ToWorkspace  VariableName=audit__mech__engine__crankshaft_KE_kJ  SampleTime=-1
  Mech Energy Nm radps : Subsystem  TreatAsAtomicUnit=on
  Mult : Product  Inputs=**
  Square : Math  Operator=square
  energy_to_workspace : ToWorkspace  VariableName=audit__mech__engine__crankshaft_kJ  SampleTime=-1
  inertia_to_workspace : ToWorkspace  VariableName=audit__mech__engine__crankshaft_kgm2  SampleTime=-1
  neg_energy_to_workspace : ToWorkspace  VariableName=audit__mech__engine__crankshaft_neg_kJ  SampleTime=-1
  one half : Gain  Gain=0.5/1000
  pos_energy_to_workspace : ToWorkspace  VariableName=audit__mech__engine__crankshaft_pos_kJ  SampleTime=-1
  power_to_workspace : ToWorkspace  VariableName=audit__mech__engine__crankshaft_kW  SampleTime=-1
  speed_to_workspace : ToWorkspace  VariableName=audit__mech__engine__crankshaft_radps  SampleTime=-1
  torque_to_workspace : ToWorkspace  VariableName=audit__mech__engine__crankshaft_Nm  SampleTime=-1
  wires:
  " trq_Nm"/1 -> torque_to_workspace/1, Mech Energy Nm radps/1(trq_Nm)
  spd_radps/1 -> Square/1, speed_to_workspace/1, Mech Energy Nm radps/2(spd_radps)
  iner_kgm2/1 -> Mult/2, inertia_to_workspace/1
  Mech Energy Nm radps/1("total_kJ ") -> energy_to_workspace/1
  Mech Energy Nm radps/4(pwr_kW) -> power_to_workspace/1
  Mech Energy Nm radps/2("pos_kJ ") -> pos_energy_to_workspace/1
  Mech Energy Nm radps/3(neg_kJ) -> neg_energy_to_workspace/1
  one half/1 -> KE_to_workspace/1
  Square/1 -> Mult/1
  Mult/1 -> one half/1

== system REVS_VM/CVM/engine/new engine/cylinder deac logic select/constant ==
  system_bus : Inport
  Constant : Constant  Value=engine.deac_strategy.enable_norm
  cyl_deac_norm : Outport
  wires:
  Constant/1 -> cyl_deac_norm/1

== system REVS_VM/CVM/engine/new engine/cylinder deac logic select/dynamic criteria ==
  system_bus : Inport
  Data Type Conversion : DataTypeConversion  OutDataTypeStr=boolean
  Data Type Conversion1 : DataTypeConversion  OutDataTypeStr=boolean
  Data Type Conversion2 : DataTypeConversion  OutDataTypeStr=double
  Latch : Subsystem
  dynamic equation : Subsystem
  dynamic equation1 : Subsystem
  cyl_deac_norm : Outport
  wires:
  Data Type Conversion2/1 -> cyl_deac_norm/1
  Data Type Conversion1/1 -> Latch/2(Off)
  Data Type Conversion/1 -> Latch/1(On)
  Latch/1(State) -> Data Type Conversion2/1
  dynamic equation1/1(out) -> Data Type Conversion1/1
  dynamic equation/1(out) -> Data Type Conversion/1
  system_bus/1 -> dynamic equation/1(bus), dynamic equation1/1(bus)

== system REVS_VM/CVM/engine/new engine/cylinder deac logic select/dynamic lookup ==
  system_bus : Inport
  Constant : Constant  Value=engine.deac_strategy.output_digital_bool
  Relay : Relay  OnSwitchValue=engine.deac_strategy.enable_threshold  OffSwitchValue=engine.deac_strategy.disable_threshold
  Switch : Switch  Criteria=u2 > Threshold
  dynamic lookup : Subsystem
  cyl_deac_norm : Outport
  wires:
  Constant/1 -> Switch/2
  Relay/1 -> Switch/1
  Switch/1 -> cyl_deac_norm/1
  dynamic lookup/1(out) -> Switch/3, Relay/1
  system_bus/1 -> dynamic lookup/1(bus)

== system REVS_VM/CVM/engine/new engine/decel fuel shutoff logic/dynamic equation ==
  bus : Inport
  Bus Creator : BusCreator  Inputs=10
  Bus Creator1 : BusCreator  Inputs=2
  Bus Selector : BusSelector  OutputSignals=var_sigs.var_sig1  OutputAsBus=on
  Data Type Conversion : DataTypeConversion  OutDataTypeStr=double
  Display : Display
  Fcn : Fcn
  Variable {1..10} (10 alike) : Constant  Value=nan
  out : Outport
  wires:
  Data Type Conversion/1 -> Fcn/1
  Bus Selector/1 -> Data Type Conversion/1, Display/1
  Bus Creator1/1 -> Bus Selector/1
  Fcn/1 -> out/1
  bus/1 -> Bus Creator1/1  "system_bus"
  Bus Creator/1 -> Bus Creator1/2  "var_sigs"
  Variable 1/1 -> Bus Creator/1  "var_sig1"
  Variable 2/1 -> Bus Creator/2  "var_sig2"
  Variable 3/1 -> Bus Creator/3  "var_sig3"
  Variable 4/1 -> Bus Creator/4  "var_sig4"
  Variable 5/1 -> Bus Creator/5  "var_sig5"
  Variable 6/1 -> Bus Creator/6  "var_sig6"
  Variable 7/1 -> Bus Creator/7  "var_sig7"
  Variable 8/1 -> Bus Creator/8  "var_sig8"
  Variable 9/1 -> Bus Creator/9  "var_sig9"
  Variable 10/1 -> Bus Creator/10  "var_sig10"

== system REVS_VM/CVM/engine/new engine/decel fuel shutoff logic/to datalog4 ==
  Var : Inport
  Constant : Constant  Value=VerboseSignal
  Constant1 : Constant  Value=VerboseLevel
  Relational Operator : RelationalOperator  OutDataTypeStr=boolean  ZeroCross=off
  Subsystem : Subsystem
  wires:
  Constant1/1 -> Relational Operator/2
  Constant/1 -> Relational Operator/1
  Relational Operator/1 -> Subsystem/Enable
  Var/1 -> Subsystem/1(In1)
